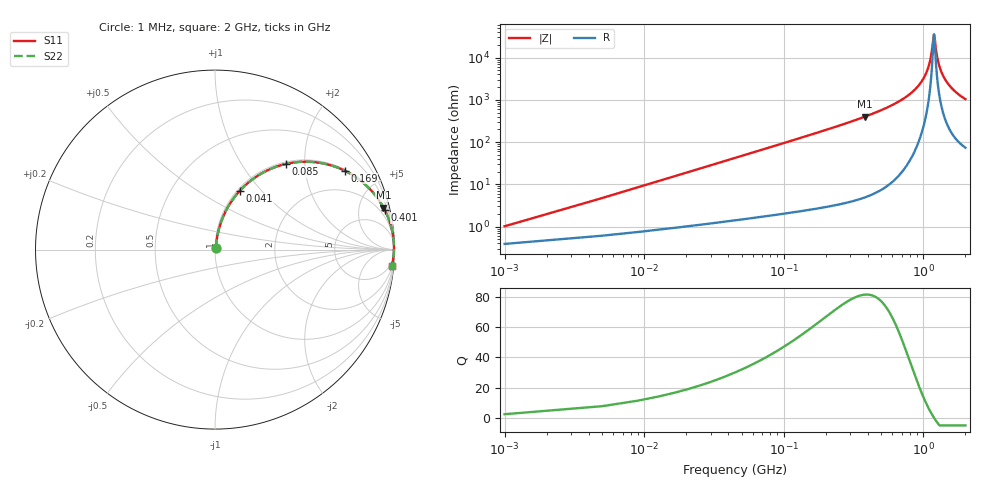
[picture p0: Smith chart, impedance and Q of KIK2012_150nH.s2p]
!version-2
!date-01.2022
!Series
# MHz S RI R 50
!Freq ReS11 ImS11 ReS21 ImS21 ReS12 ImS12 ReS22 ImS22
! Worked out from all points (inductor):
!   501 points, 1 MHz to 2 GHz, reference 50 ohm
!   read as one part in series: L = 150 nH near 9 MHz
!   highest Q = 81.4 at 381 MHz (marker M1), where L = 167 nH
!   self-resonance near 1.189 GHz
!   S11 on the Smith chart (normalised r, x): 1 MHz: 1.01, +0.02; 41 MHz: 1.03, +0.77; 85 MHz: 1.04, +1.61; 169 MHz: 1.05, +3.25; 401 MHz: 1.10, +8.52; 2 GHz: 2, -21
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1  0.00397 0.00935  0.996 -0.00935  0.996 -0.00935  0.00397 0.00935
13  0.0229 0.1187  0.9771 -0.1187  0.9771 -0.1187  0.0229 0.1187
17  0.0337 0.1534  0.9663 -0.1534  0.9663 -0.1534  0.0337 0.1534
29  0.0789 0.249  0.9211 -0.249  0.9211 -0.249  0.0789 0.249
41  0.1388 0.3287  0.8612 -0.3287  0.8612 -0.3287  0.1388 0.3287
85  0.3958 0.4775  0.6042 -0.4775  0.6042 -0.4775  0.3958 0.4775
169  0.7223 0.4398  0.2777 -0.4398  0.2777 -0.4398  0.7223 0.4398
337  0.9198 0.2655  0.0802 -0.2655  0.0802 -0.2655  0.9198 0.2655
381  0.9386 0.2339  0.0614 -0.2339  0.0614 -0.2339  0.9386 0.2339
401  0.9454 0.2212  0.0546 -0.2212  0.0546 -0.2212  0.9454 0.2212
669  0.9865 0.107  0.0135 -0.107  0.0135 -0.107  0.9865 0.107
869  0.9947 0.0568  0.00528 -0.0568  0.00528 -0.0568  0.9947 0.0568
1001  0.9967 0.0311  0.00325 -0.0311  0.00325 -0.0311  0.9967 0.0311
1113  0.9973 0.0122  0.00273 -0.0122  0.00273 -0.0122  0.9973 0.0122
1145  0.9973 0.00717  0.00273 -0.00717  0.00273 -0.00717  0.9973 0.00717
1181  0.9972 0.00169  0.00279 -0.00169  0.00279 -0.00169  0.9972 0.00169
1193  0.9972 -0.000101  0.00283 0.000101  0.00283 0.000101  0.9972 -0.000101
1257  0.9969 -0.00934  0.00313 0.00934  0.00313 0.00934  0.9969 -0.00934
1337  0.9962 -0.0203  0.00376 0.0203  0.00376 0.0203  0.9962 -0.0203
1469  0.9947 -0.037  0.00528 0.037  0.00528 0.037  0.9947 -0.037
1669  0.9915 -0.0601  0.00851 0.0601  0.00851 0.0601  0.9915 -0.0601
2000  0.9843 -0.0939  0.0157 0.0939  0.0157 0.0939  0.9843 -0.0939
